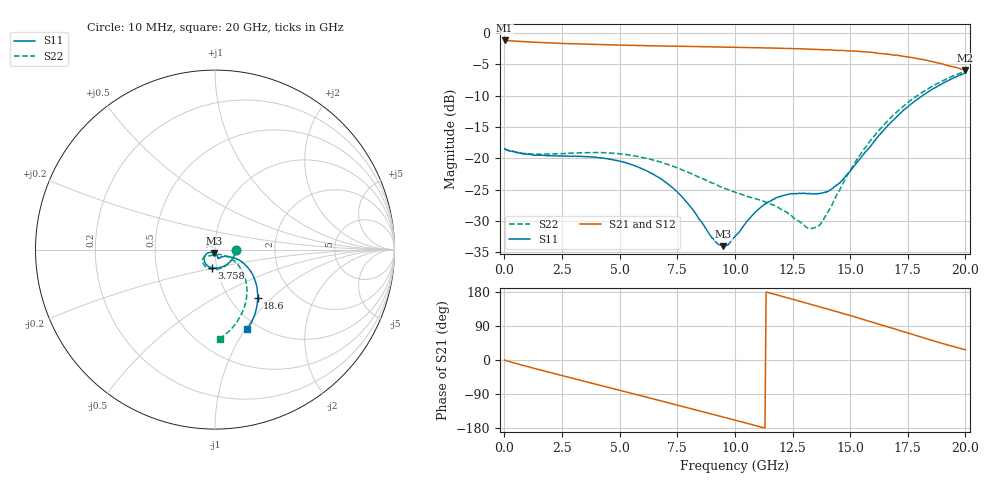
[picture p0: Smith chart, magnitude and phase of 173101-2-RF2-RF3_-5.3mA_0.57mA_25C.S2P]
!  2-Port S-parameters saved by WinCal
! VAR MeasName=S-Parameters (CALIBRATED_DATA) read from VNA (N5242A)
! VAR MeasDate=2017-7-20 9:30:19
! VAR NAME=173101-2-RF2-RF3_-5.3mA_0.57mA_25C
! VAR FILENAME=173101-2-RF2-RF3_-5.3mA_0.57mA_25C.S2P
! VAR DATE=2017-7-20 9:30:19
! VAR PHYS_PORTS=1,2
# Hz S DB R 50
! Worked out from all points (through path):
!   401 points, 10 MHz to 20 GHz, reference 50 ohm
!   highest |S21| = -1.19 dB at 10 MHz (marker M1); lowest = -5.9 dB at 20 GHz (marker M2)
!   group delay of S21, straight-line fit = 45.8 ps
!   lowest |S11| = -34.0 dB at 9.505 GHz (marker M3), VSWR 1.04, Z = 49.3 - j1.83 ohm
!   |S11| at or under -10 dB: start of sweep to 18.13 GHz
!   |S22| runs from -31.2 to -6.1 dB; largest |S21 - S12| = 0.0085
!   S11 on the Smith chart (normalised r, x): 10 MHz: 1.27, -0.00; 3.758 GHz: 0.94, -0.19; 18.6 GHz: 1.33, -0.82; 20 GHz: 0.88, -1.02
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1e7  -18.48 -0.7  -1.19 -0.2  -1.19 -0.2  -18.45 -0.7
1.559225e9  -19.48 -51.1  -1.51 -26.4  -1.52 -26.3  -19.31 -51.4
3.358325e9  -19.68 -92.9  -1.78 -54.5  -1.78 -54.5  -19.10 -91.8
3.758125e9  -19.76 -100.8  -1.82 -60.7  -1.82 -60.7  -19.07 -98.9
5.2074e9  -20.63 -125.9  -1.96 -83.2  -1.97 -83.0  -19.35 -121.0
6.70665e9  -23.06 -146.5  -2.06 -106.5  -2.06 -106.3  -20.50 -137.6
8.006e9  -27.40 -154.7  -2.13 -126.8  -2.16 -126.7  -22.29 -145.5
9.0055e9  -32.70 -137.1  -2.20 -142.5  -2.21 -142.3  -23.92 -145.5
9.50525e9  -34.00 -111.1  -2.25 -150.6  -2.24 -150.5  -24.74 -143.6
1.0005e10  -32.45 -86.9  -2.29 -158.6  -2.29 -158.5  -25.39 -140.2
1.085458e10  -28.66 -70.5  -2.34 -172.3  -2.35 -172.2  -26.40 -134.0
1.145428e10  -26.92 -69.6  -2.39 177.8  -2.40 178.0  -27.12 -129.0
1.230385e10  -25.75 -70.9  -2.47 163.7  -2.47 163.9  -28.74 -119.1
1.310345e10  -25.58 -66.0  -2.57 150.2  -2.57 150.4  -31.01 -96.5
1.335332e10  -25.69 -63.2  -2.60 146.0  -2.58 146.3  -31.13 -83.1
1.375312e10  -25.59 -55.4  -2.66 139.1  -2.66 139.3  -30.25 -60.2
1.455272e10  -23.94 -36.3  -2.77 125.4  -2.76 125.6  -24.99 -32.8
1.575212e10  -18.62 -23.7  -3.04 103.5  -3.04 103.8  -17.81 -31.3
1.670165e10  -14.54 -26.8  -3.40 86.1  -3.45 86.1  -13.75 -40.0
1.76012e10  -11.47 -35.7  -3.87 69.6  -3.87 69.9  -10.82 -51.7
1.86007e10  -8.89 -48.5  -4.61 50.9  -4.65 51.3  -8.42 -66.2
2e10  -6.39 -68.1  -5.90 26.8  -5.95 27.6  -6.09 -86.9
